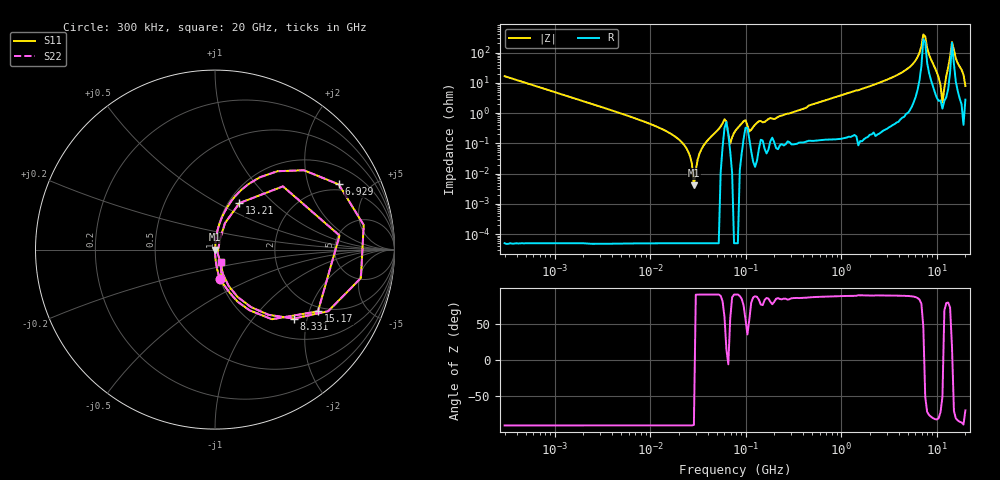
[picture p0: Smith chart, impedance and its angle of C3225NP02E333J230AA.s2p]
! S-parameter Generated by TDK Corporation
! Copyright(C) 2015 TDK Corporation.
! All Rights Reserved.
! TDK P/N: C3225NP02E333J230AA (Multilayer Ceramic Chip Capacitors)
! Property: C=33nF
! Size(LxWxT): 3.2x2.5x2.3mm, 0.126x0.098x0.091inches
! Model Type: s2p (Touchstone File Format Version 1.0)
! Frequency: DC=Yes Start=0.3MHz Stop=20000MHz 243points Log-sweep
! Note:
! Model Generated on Jun. 23, 2015
! Hash(MD5):
! Port Assignments:
!  1 ---| |--- 2
! Applicable Conditions:
!  Temperature = 25 degC
!  DC Bias Voltage = 0 V
!  Small Signal Operation
! Terms and conditions regarding TDK Simulation Models
! (1)This simulation model is being provided solely for informational purposes. Please refer to the specifications of the products in terms of detailed characteristics of such products.
! (2)In no event shall TDK Corporation of any of its subsidiaries be liable for any loss or damage arising, directly or indirectly,
!  From any information contained in this simulation model, including, but not limited to loss or damages arising from any inaccuracies, omissions or errors in connection with such information.
! (3)Any and all copyrights on this simulation model are owned by TDK Corporation.
!  Duplication or redistribution of this simulation model without prior written permission from TDK Corporation is prohibited.
! (4)This simulation model is subject to any modification or change without any prior notice.
! (5)Neither TDK Corporation nor any of its subsidiaries shall make any warranty, express or implied,
!  Including but not limited to the correctness, implied warranties of merchantability and fitness for a particular purpose with respect to this simulation models.
! (6)The use of this simulation model shall be deemed to have consented to the terms and conditions hereof.
# MHz S MA R 50
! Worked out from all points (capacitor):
!   242 points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, 300 kHz to 20 GHz, reference 50 ohm
!   read as one part in series: C = 32 nF near 314.2 kHz
!   lowest |Z| = 4.09 mohm at 28.76 MHz (marker M1)
!   series resonance near 29.08 MHz, so ESL is about 940 pH
!   S11 on the Smith chart (normalised r, x): 300 kHz: 1.00, -0.33; 6.929 GHz: 1.72, +3.18; 8.331 GHz: 1.42, -1.66; 13.21 GHz: 1.12, +0.64; 15.17 GHz: 1.84, -2.29; 20 GHz: 1.06, -0.15
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0.3  0.1634 -80.6  0.9866 9.4  0.9866 9.4  0.1634 -80.6
1.985118  0.02492 -88.6  0.9997 1.4  0.9997 1.4  0.02492 -88.6
12.54397  0.003257 -92.7  0.9998 0.2  0.9998 0.2  0.003257 -92.7
21.80869  0.001046 -99.4  0.9998 0.1  0.9998 0.1  0.001046 -99.4
28.7559  0.000182 -167.0  0.9998 0.0  0.9998 0.0  0.000182 -167.0
60.11549  0.006278 59.3  0.9968 -0.3  0.9968 -0.3  0.006278 59.3
69.02956  0.0009868 57.5  0.9995 -0.0  0.9995 -0.0  0.0009868 57.5
79.26541  0.002751 90.5  1 -0.2  1 -0.2  0.002751 90.5
99.80788  0.005839 55.4  0.9967 -0.3  0.9967 -0.3  0.005839 55.4
500.8786  0.01939 85.3  0.9986 -1.1  0.9986 -1.1  0.01939 85.3
3165.055  0.1336 80.9  0.9877 -7.7  0.9877 -7.7  0.1336 80.9
5502.7  0.3577 66.6  0.9188 -20.9  0.9188 -20.9  0.3577 66.6
6928.783  0.7792 27.8  0.4772 -49.5  0.4772 -49.5  0.7792 27.8
7255.597  0.8397 9.4  0.2114 -35.8  0.2114 -35.8  0.8397 9.4
8331.474  0.583 -41.3  0.6796 34.4  0.6796 34.4  0.583 -41.3
10490.66  0.1441 -72.1  0.9654 8.2  0.9654 8.2  0.1441 -72.1
11503.64  0.02269 -51.4  0.986 0.9  0.986 0.9  0.02269 -51.4
13209.43  0.2931 62.2  0.901 -16.7  0.901 -16.7  0.2931 62.2
14484.93  0.6983 6.5  0.3117 -11.0  0.3117 -11.0  0.6983 6.5
15168.15  0.6689 -31.0  0.5473 38.9  0.5473 38.9  0.6689 -31.0
19099.14  0.1835 -78.2  0.979 10.6  0.979 10.6  0.1835 -78.2
20000  0.0765 -65.1  0.9703 4.1  0.9703 4.1  0.0765 -65.1
